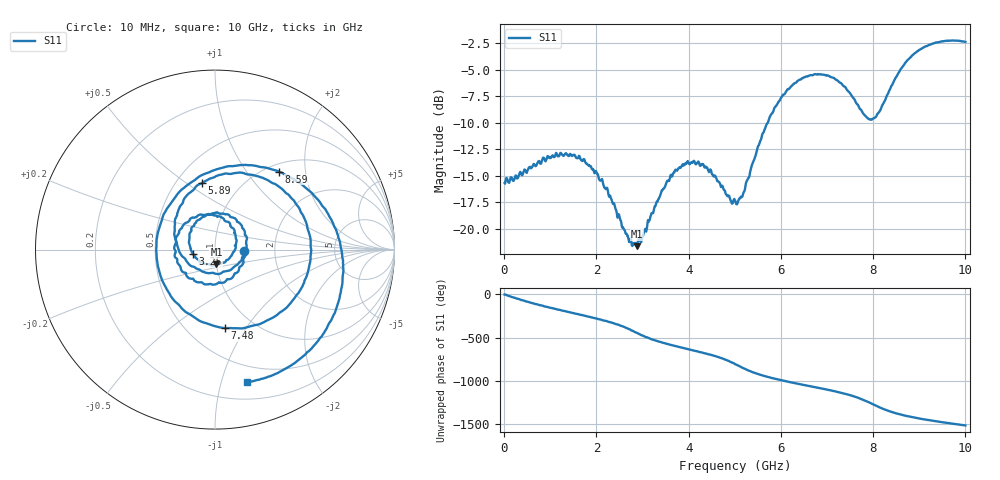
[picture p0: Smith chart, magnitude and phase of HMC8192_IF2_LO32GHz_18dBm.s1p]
! Analog Devices, Inc.
! 1 Analog Way
! Wilmington, MA 01887
! http://www.analog.com
! Date:  2021-09-17 NN
! Board Name:  EVALHMC8192LG Revision A with HMC8192LG installed
! File Description:  S-Parameters for evaluation board without connectors or board loss de-embedded
! File Generation:  Calibrated Network Analyzer
! Chip Part Number:  HMC8192
! Chip Description:  Wideband IQ Mixer
! Chip Frequency:  20 to 42 GHz
! Chip Package:  LGA_CAV, 4 x 4 x 1.55 mm
! Chip State:
!  Temperature:  25C
!  LO Frequency:  32GHz
!  LO Power:  18dBm
! Note:
!  Analog Devices supplies this data as a sample of measured data at the evaluation board
!  ports for this product.  Your particular data for this product may vary.
!  Analog Devices reserves the right to change this data at anytime.
!  All lines below in this file are as is from the Network Analyzer.
!Keysight Technologies,N5245A,MY49151104,A.10.65.16
!Date: Tuesday, September 14, 2021 12:22:56
!Correction: S22(Full 2 Port(1,2))
!S1P File: Measurement: S22:
# Hz S  dB  R 50
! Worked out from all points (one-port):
!   1000 points, 10 MHz to 10 GHz, reference 50 ohm
!   lowest |S11| = -21.7 dB at 2.87 GHz (marker M1), VSWR 1.18, Z = 50.1 - j8.29 ohm
!   |S11| at or under -10 dB: start of sweep to 5.717 GHz
!   S11 on the Smith chart (normalised r, x): 10 MHz: 1.39, -0.02; 3.25 GHz: 0.78, -0.04; 5.89 GHz: 0.66, +0.58; 7.48 GHz: 0.75, -0.81; 8.59 GHz: 1.13, +1.44; 10 GHz: 0.35, -1.21
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1e7  -15.70 -2.4
6e8  -14.25 -98.9
1.26e9  -13.04 171.7
1.86e9  -14.09 98.3
2.51e9  -19.03 0.4
2.87e9  -21.66 -84.5
3.25e9  -18.11 -167.7
3.76e9  -14.44 115.6
4.08e9  -13.73 73.8
4.45e9  -14.61 25.4
5.01e9  -17.39 -87.9
5.5e9  -12.28 159.1
5.89e9  -8.44 101.1
6.26e9  -6.41 57.3
6.59e9  -5.61 22.3
6.88e9  -5.46 -8.4
7.21e9  -5.98 -45.9
7.48e9  -7.11 -82.6
7.51e9  -7.29 -87.6
7.8e9  -9.23 -142.4
8.02e9  -9.58 162.9
8.32e9  -7.29 94.2
8.59e9  -5.00 50.6
8.76e9  -4.05 28.9
9.01e9  -3.11 2.5
9.3e9  -2.53 -23.3
9.68e9  -2.26 -52.4
1e10  -2.38 -76.4
